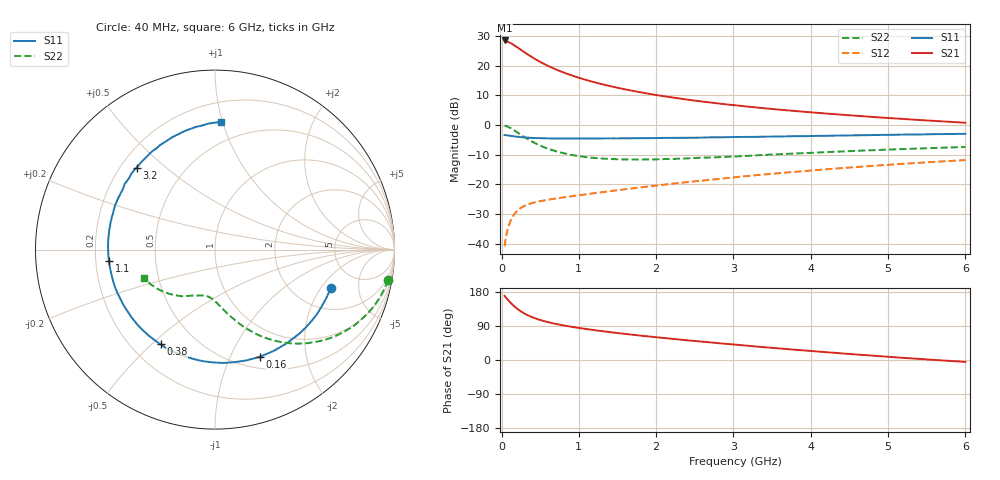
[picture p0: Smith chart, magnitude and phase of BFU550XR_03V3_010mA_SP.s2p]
! Filename:  P:\Prog\Test\Noise\ATS_data\Testdata_Net\03 Spar\BFU550XR_APG2013_45_C05_03p3V_010mA_SP_CM01_D.s2p
! Date/Time: Tue 06/Aug/2013 14:38:14
! BFU550XR_APG2013_45_C05_03p3V_1to35mA_SP_CM01_Bias5_R.s2p
! MDIF S-parameter v. bias file
! BFU550XR_APG2013_45_C05_03p3V_1to35mA_SP_CM01
! Date/time Fri Aug 02 14:41:13 2013
! VAR V_out= 3.3000
! VAR I_out= 10.0000
! VAR V_in= 0.8305
! VAR I_in= 0.1129
! Device data file deembeded for feedlines and parallel
! Original file: \03 Spar\BFU550XR_APG2013_45_C05_03p3V_010mA_SP_CM01_R.s2p
! Feed-files: PR006V01_02082013_Feed1.s2p, PR006V01_02082013_Feed2.s2p
! Parallel-file: PR006V01_02082013_Par.s2p
# MHz S MA R 50
!  Freq-MHz  S11-mag  S11-arg  S21-mag  S21-arg  S12-mag  S12-arg  S22-mag  S22-arg
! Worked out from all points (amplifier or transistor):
!   98 points, 40 MHz to 6 GHz, reference 50 ohm
!   highest |S21| = 28.5 dB at 40 MHz (marker M1)
!   |S21| within 3 dB of that: start of sweep to 242.7 MHz
!   unconditionally stable (mu >= 1): 1.882 GHz to 4.007 GHz
!   at 300 MHz: K = 0.29, MSG = 25.8 dB, |S12| = -27.2 dB
!   at 1.6 GHz: K = 0.95, MSG = 16.8 dB, |S12| = -21.6 dB
!   at 6 GHz: K = 0.88, MSG = 6.3 dB, |S12| = -11.8 dB
!   S11 on the Smith chart (normalised r, x): 40 MHz: 3.13, -2.50; 160 MHz: 0.63, -1.30; 380 MHz: 0.32, -0.53; 1.1 GHz: 0.26, -0.05; 3.2 GHz: 0.26, +0.40; 6 GHz: 0.34, +0.99
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40  0.68 -18.4  26.57 169.4  0.009151 81.6  0.977 -10.0
50  0.6767 -23.0  26.42 166.2  0.01132 79.4  0.9702 -12.6
100  0.6639 -44.5  24.65 154.9  0.02143 70.1  0.9112 -24.4
120  0.6577 -52.6  23.95 150.4  0.02491 66.6  0.8836 -28.6
160  0.6474 -67.1  22.18 142.7  0.03089 60.8  0.8219 -36.2
220  0.6332 -85.9  19.74 132.6  0.03765 54.1  0.7294 -45.6
260  0.6253 -96.2  18.15 127.1  0.04101 50.7  0.6738 -50.9
320  0.6157 -109.5  16.08 120.1  0.04497 46.8  0.6011 -57.2
380  0.6086 -119.8  14.29 114.5  0.04797 44.2  0.5414 -62.4
433  0.605 -127.7  12.98 110.2  0.05014 42.7  0.4978 -66.1
500  0.6018 -135.6  11.58 105.7  0.05248 41.3  0.4534 -70.1
650  0.5959 -149.4  9.281 97.6  0.05672 40.2  0.3815 -76.9
800  0.595 -159.4  7.705 91.4  0.06067 40.3  0.337 -82.1
1050  0.5945 -171.8  5.979 83.1  0.06712 41.8  0.2937 -88.6
1100  0.5935 -173.9  5.718 81.6  0.06849 42.1  0.2885 -89.8
1500  0.5975 172.5  4.248 71.2  0.08008 44.5  0.266 -97.5
2050  0.6055 158.2  3.132 59.1  0.09737 46.4  0.2662 -106.2
3100  0.6317 135.7  2.103 39.1  0.1357 46.3  0.2997 -120.5
3200  0.632 133.7  2.038 37.3  0.1396 46.0  0.3039 -121.7
4100  0.6581 117.5  1.601 22.2  0.1759 42.2  0.3456 -133.6
5200  0.691 99.2  1.267 5.6  0.2233 35.3  0.3946 -147.8
6000  0.7128 87.1  1.095 -5.0  0.2571 29.1  0.4278 -158.3
